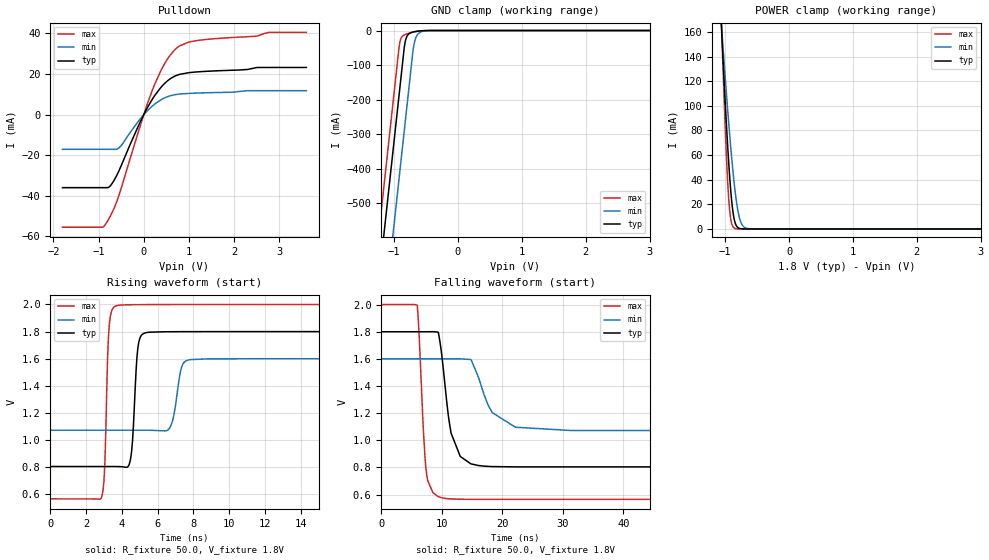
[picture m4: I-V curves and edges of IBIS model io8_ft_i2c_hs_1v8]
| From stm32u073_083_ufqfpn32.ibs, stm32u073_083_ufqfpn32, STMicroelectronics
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[Model]   io8_ft_i2c_hs_1v8
Model_type I/O_open_drain
Polarity   Non-Inverting
Enable   Active-Low
| CAP_THRESHOLD on pad IOFT is "UDTCAPC" :
| Rising=30.0% of vddiom   Falling=70.0% of vddiom
| C_comp min and max val. don't necessarily correlate with the min and max pvt
| but are the smallest and greatest pad capacitance found.
| var   typ   min   max
C_comp   2.35140pF  2.33125pF  2.40370pF
|C_comp_pulldown   2.35140pF  2.33125pF  2.40370pF
Vinl = 800.0mV
Vinh = 1.0V
Vmeas = 900.0mV   | Reference voltage for timing measurements
Cref  = 50.0pF   | Timing specification test load capacitance value
Rref  = 1.0MOhm   | Timing specification test load resistance value
Vref  = 990.0mV   | Timing specification test load voltage
[Model Spec]
| TIME_THRESHOLD on pin ZIV12 is "CMOS" :
| Rising=50.0% of vdd   Falling=50.0% of vdd
Vinl 728.70000mV 652.70000mV 817.70000mV
Vinh 1.06430V 953.30000mV 1.16330V
| variable   typ   min   max
[Temperature Range] 25.0 125.0 -40.0
| variable   typ   min   max
[Voltage Range] 1.8V 1.6V 2.0V
| variable   typ   min   max
[POWER Clamp Reference] 1.8V 1.6V 2.0V
| variable   typ   min   max
[GND Clamp Reference] 0V 0V 0V
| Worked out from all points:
|   slope of the pulldown table from 0 to 0.27 V, typ, clamps not added: 26.4 ohm
|   GND clamp passes 1 mA (typ) near -0.58 V on its own axis
|   POWER clamp passes 1 mA (typ) near -0.80 V on its own axis
|   rising waveform, R_fixture 50.0, V_fixture 1.8V: 20-80 % time 239ps typ, 366ps min, 181ps max; typ from 0.804 V to 1.8 V
|   falling waveform, R_fixture 50.0, V_fixture 1.8V: 20-80 % time 1.91ns typ, 3.49ns min, 942ps max; typ from 1.8 V to 0.804 V
[POWER Clamp]
-1.8V     1.076A     768.4mA    1.428A
-1.06V    166.8mA    167.3mA    172.4mA
-1.05V    156mA      159.9mA    156.7mA
-990mV    94.58mA    117mA      71.25mA
-950mV    58.69mA    90.08mA    29.27mA
-930mV    43.17mA    77.3mA     15.67mA
-910mV    29.83mA    65.11mA    7.377mA
-860mV    8.434mA    38.02mA    795.5uA
-810mV    1.577mA    17.81mA    74.4uA
-770mV    365.4uA    7.942mA    11.04uA
-650mV    4.138uA    347.7uA    35.9nA
3.6V      0A         0A         0A
[GND Clamp]
-1.8V     -1.68A     -1.921A    -1.54A
-1.24V    -727.6mA   -969.1mA   -588.3mA
-1.05V    -404.6mA   -646.1mA   -265.3mA
-920mV    -183.6mA   -425.1mA   -45.19mA
-890mV    -132.6mA   -374.1mA   -22.26mA
-850mV    -64.62mA   -306.1mA   -13.71mA
-830mV    -36.28mA   -272.1mA   -11.85mA
-800mV    -17.27mA   -221.1mA   -9.806mA
-690mV    -3.766mA   -41.92mA   -4.242mA
-640mV    -2.189mA   -13.56mA   -2.404mA
-570mV    -808.8uA   -3.218mA   -757.3uA
3.6V      453.9pA    48.38nA    315.2pA
| variable   typ   min   max
[Pullup Reference] 1.8V 1.6V 2.0V
| variable   typ   min   max
[Pulldown Reference] 0V 0V 0V
[Pulldown]
-1.8V     -35.95mA   -17.07mA   -55.42mA
-910mV    -35.95mA   -17.07mA   -55.42mA
-830mV    -35.95mA   -17.07mA   -53.41mA
-720mV    -34.49mA   -17.07mA   -49.08mA
-540mV    -27.18mA   -16.22mA   -39.07mA
-120mV    -5.598mA   -3.255mA   -8.496mA
240mV     9.353mA    5.171mA    14.85mA
490mV     15.96mA    8.523mA    26.14mA
750mV     19.54mA    10.04mA    33.17mA
1.37V     21.33mA    10.77mA    37.03mA
2.78V     23.25mA    11.81mA    40.55mA
3.6V      23.25mA    11.81mA    40.56mA
[Ramp]
dV/dt_r 597.4203mV/236.95104ps 316.60858mV/363.82074ps 860.75297mV/176.73075ps
dV/dt_f 597.45872mV/1.71663ns 316.65389mV/2.97475ns 860.78191mV/941.93765ps
R_load = 50.0
| Removed startup time: 0s 0s 0s  .
| Removed end time: 19.75ns.
[Rising Waveform]
R_fixture   = 50.0
V_fixture   = 1.8V
V_fixture_min = 1.6V
V_fixture_max = 2.0V
0s        804.2mV    1.072V     565.4mV
2.9ns     804mV      1.072V     591mV
3.25ns    804mV      1.072V     1.754V
3.6ns     804mV      1.072V     1.985V
4.45ns    835.5mV    1.072V     1.998V
4.9ns     1.682V     1.072V     1.999V
5.25ns    1.788V     1.072V     1.999V
6.7ns     1.799V     1.094V     2V
7.7ns     1.799V     1.589V     2V
19.75ns   1.8V       1.6V       2V
| Removed startup time: 0s 0s 0s  .
| Removed end time: 99.775ns.
[Falling Waveform]
R_fixture   = 50.0
V_fixture   = 1.8V
V_fixture_min = 1.6V
V_fixture_max = 2.0V
0s        1.8V       1.6V       2V
5.925ns   1.8V       1.6V       1.993V
7.45ns    1.8V       1.6V       764.5mV
9.825ns   1.686V     1.6V       578.8mV
11.53ns   1.054V     1.6V       568.2mV
13.05ns   881.2mV    1.6V       566mV
16.02ns   814.6mV    1.469V     565.4mV
18.35ns   806.6mV    1.204V     565.4mV
22.18ns   804.4mV    1.097V     565.4mV
99.78ns   804.2mV    1.072V     565.4mV
